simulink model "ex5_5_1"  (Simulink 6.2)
settings: Solver=ode45  SolverMode=SingleTasking  StartTime=0.0  StopTime=1000  MaxStep=10  RelTol=1e-3  AbsTol=1e-6

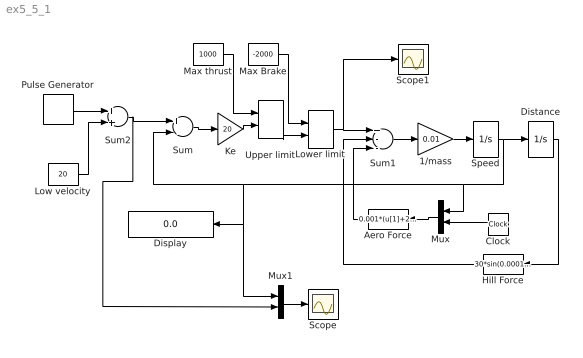
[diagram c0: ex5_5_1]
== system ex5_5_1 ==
  1/mass : Gain  Gain=0.01
  Aero Force : Fcn  Orientation=left  Expr=0.001*(u[1]+20*sin(0.01*u[2]))^2
  Clock : Clock
  Display : Display
  Distance : Integrator
  Hill Force : Fcn  Orientation=left  Expr=30*sin(0.0001*u[1])
  Ke : Gain  Gain=20
  Low velocity : Constant  Value=20
  Lower limit : MinMax  Function=max  Inputs=2
  Max Brake : Constant  Value=-2000
  Max thrust : Constant  Value=1000
  Mux : Mux  Orientation=left  Inputs=2
  Mux1 : Mux  Inputs=2
  Pulse Generator : DiscretePulseGenerator  PulseType=Time based  Amplitude=40  Period=500  PulseWidth=50
  Scope : Scope
  Scope1 : Scope
  Speed : Integrator
  Sum : Sum  Inputs=+-
  Sum1 : Sum  Inputs=+--
  Sum2 : Sum
  Upper limit : MinMax  Inputs=2
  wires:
  Speed/1 -> Distance/1, Mux/1, Sum/2, Display/1, Mux1/1
  Sum/1 -> Ke/1
  Mux/1 -> Aero Force/1
  Aero Force/1 -> Sum1/3
  Hill Force/1 -> Sum1/2
  Distance/1 -> Hill Force/1
  Sum1/1 -> 1/mass/1
  1/mass/1 -> Speed/1
  Ke/1 -> Upper limit/2
  Upper limit/1 -> Lower limit/2
  Max thrust/1 -> Upper limit/1
  Max Brake/1 -> Lower limit/1
  Clock/1 -> Mux/2
  Lower limit/1 -> Sum1/1, Scope1/1
  Pulse Generator/1 -> Sum2/1
  Sum2/1 -> Sum/1, Mux1/2
  Low velocity/1 -> Sum2/2
  Mux1/1 -> Scope/1
